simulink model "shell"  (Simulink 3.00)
settings: Solver=ode45  SolverMode=SingleTasking  StartTime=0.0  StopTime=999999  RelTol=1e-3  AbsTol=1e-6
undefined symbols (not defined in the file or in its folder): Manual

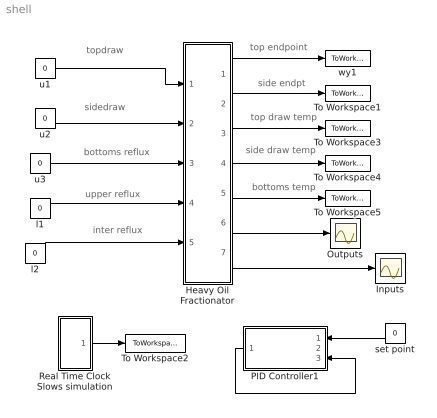
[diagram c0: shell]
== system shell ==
  note: topdraw
  note: sidedraw
  note: bottoms reflux
  note: upper reflux
  note: inter reflux
  note: top endpoint
  note: side endpt
  note: top draw temp
  note: side draw temp
  note: bottoms temp
  Heavy Oil Fractionator : Subsystem  mask{e5=0.0, e4=0.0, e3=0.0, e2=0.0, e1=0.0}
      mask prompts: e5 "Error in Upp Ref Duty Tfns"; e4 "Error in Int Ref Duty Tfns"; e3 "Error in Bott duty tfns"; e2 "Err in Side draw tfns"; e1 "Error in top draw tfs"
      mask init:
      | e1=0;e2=0;e3=0;e4=0;e5=0;
  Inputs : Scope
  Outputs : Scope
  PID Controller1 : Subsystem  Orientation=left  mask(Real PID Controller){am_flag=Manual, co=0, Ts=1, Kc=0, taui=999999, taud=0, co_max=.5, co_min=-.5, al=0}
      mask prompts: am_flag "Auto/Manual Switch"; co "Manual Controller Output"; Ts "Sample Time,Ts"; Kc "Kc: Proportional Gain: Negative for DIRECT Action"; taui "taui: Integral time"; taud "Derivative Time, taud"; co_max "Upper limit for controller output"; co_min "Lower limit for controller output"; al "Noise filter tim const, al"
      mask help: Programmed by Babu Joseph, Washington Universtiy in St. Louis, 1998
  Real Time Clock Slows simulation : Subsystem  mask(Sample time){Ts=1}
      mask prompts: Ts "Sample time"
      mask help: This block is used to set the sample time.
  To Workspace1 : ToWorkspace  VariableName=y2  SampleTime=1  SaveFormat=Matrix
  To Workspace2 : ToWorkspace  VariableName=t  SampleTime=1  SaveFormat=Matrix
  To Workspace3 : ToWorkspace  VariableName=y3  SampleTime=1  SaveFormat=Matrix
  To Workspace4 : ToWorkspace  VariableName=y5  SampleTime=1  SaveFormat=Matrix
  To Workspace5 : ToWorkspace  VariableName=y7  SampleTime=1  SaveFormat=Matrix
  l1 : Constant  Value=0
  l2 : Constant  Value=0
  set point : Constant  Orientation=left  Value=0
  u1 : Constant  Value=0
  u2 : Constant  Value=0
  u3 : Constant  Value=0
  wy1 : ToWorkspace  VariableName=y1  SampleTime=1  SaveFormat=Matrix
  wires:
  u3/1 -> Heavy Oil Fractionator/3(u3)
  l2/1 -> Heavy Oil Fractionator/5(l2)
  l1/1 -> Heavy Oil Fractionator/4(l1)
  Heavy Oil Fractionator/6(outputs) -> Outputs/1
  Heavy Oil Fractionator/7(inputs) -> Inputs/1
  Heavy Oil Fractionator/2(y2) -> To Workspace1/1
  Heavy Oil Fractionator/3(y3) -> To Workspace3/1
  Heavy Oil Fractionator/4(y5) -> To Workspace4/1
  Heavy Oil Fractionator/5(y7) -> To Workspace5/1
  Real Time Clock Slows simulation/1("Clock ") -> To Workspace2/1
  u2/1 -> Heavy Oil Fractionator/2(u2)
  Heavy Oil Fractionator/1(y1) -> wy1/1
  u1/1 -> Heavy Oil Fractionator/1(u1)
  set point/1 -> PID Controller1/1(setpt)
  PID Controller1/1(output) -> PID Controller1/3(out_fdbk)
  ? -> PID Controller1/2(meas)

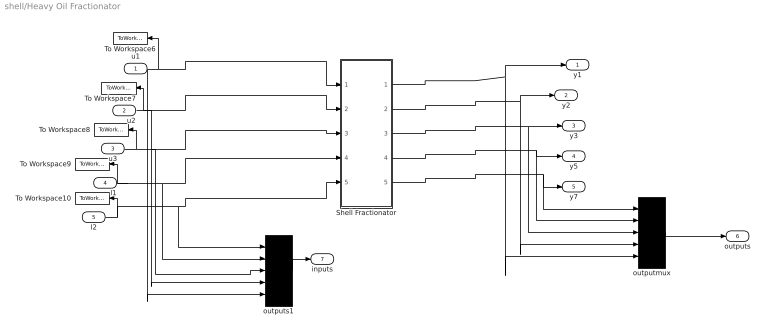
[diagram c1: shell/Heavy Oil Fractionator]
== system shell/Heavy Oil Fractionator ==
  u1 : Inport  Port=1  PortWidth=-1  SampleTime=-1  DataType=auto
  u2 : Inport  Port=2  PortWidth=-1  SampleTime=-1  DataType=auto
  u3 : Inport  Port=3  PortWidth=-1  SampleTime=-1  DataType=auto
  l1 : Inport  Port=4  PortWidth=-1  SampleTime=-1  DataType=auto
  l2 : Inport  Port=5  PortWidth=-1  SampleTime=-1  DataType=auto
  Shell Fractionator : Subsystem
  To Workspace10 : ToWorkspace  VariableName=l2  SampleTime=1  SaveFormat=Matrix
  To Workspace6 : ToWorkspace  VariableName=u1  SampleTime=1  SaveFormat=Matrix
  To Workspace7 : ToWorkspace  VariableName=u2  SampleTime=1  SaveFormat=Matrix
  To Workspace8 : ToWorkspace  VariableName=u3  SampleTime=1  SaveFormat=Matrix
  To Workspace9 : ToWorkspace  VariableName=l1  SampleTime=1  SaveFormat=Matrix
  outputmux : Mux  Inputs=5
  outputs1 : Mux  Inputs=5
  y1 : Outport  Port=1  InitialOutput=0
  y2 : Outport  Port=2  InitialOutput=0
  y3 : Outport  Port=3  InitialOutput=0
  y5 : Outport  Port=4  InitialOutput=0
  y7 : Outport  Port=5  InitialOutput=0
  outputs : Outport  Port=6  InitialOutput=0
  inputs : Outport  Port=7  InitialOutput=0
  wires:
  l2/1 -> To Workspace10/1, outputs1/1, Shell Fractionator/5(l2)
  l1/1 -> To Workspace9/1, outputs1/2, Shell Fractionator/4(l1)
  u3/1 -> To Workspace8/1, outputs1/3, Shell Fractionator/3(u3)
  u2/1 -> To Workspace7/1, outputs1/4, Shell Fractionator/2(u2)
  outputmux/1 -> outputs/1
  outputs1/1 -> inputs/1
  u1/1 -> To Workspace6/1, Shell Fractionator/1(u1), outputs1/5
  Shell Fractionator/1(y1) -> y1/1, outputmux/5
  Shell Fractionator/2(y2) -> y2/1, outputmux/4
  Shell Fractionator/3(y3) -> y3/1, outputmux/3
  Shell Fractionator/4(y5) -> y5/1, outputmux/2
  Shell Fractionator/5(y7) -> y7/1, outputmux/1

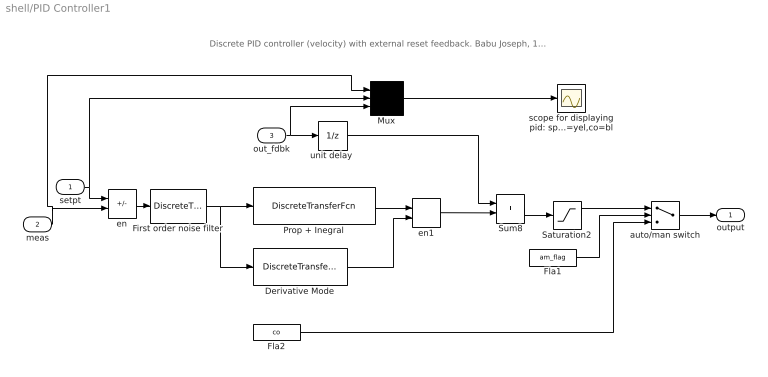
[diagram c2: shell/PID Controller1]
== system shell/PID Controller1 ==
  note: Discrete PID controller (velocity) with external reset feedback. Babu Joseph, 1998
  setpt : Inport  Port=1  PortWidth=-1  SampleTime=-1  DataType=auto
  meas : Inport  Port=2  PortWidth=-1  SampleTime=-1  DataType=auto
  out_fdbk : Inport  Port=3  PortWidth=-1  SampleTime=-1  DataType=auto
  Derivative Mode : DiscreteTransferFcn  Numerator=Kc*taud*[1 -2 1]  Denominator=[ 1 0 0]  SampleTime=Ts
  First order noise filter : DiscreteTransferFcn  Numerator="[Ts   0]"  Denominator="[(al+Ts)  -al]"  SampleTime=Ts
  Fla1 : Constant  Value=am_flag
  Fla2 : Constant  Value=co
  Mux : Mux  Inputs=3
  Prop + Inegral : DiscreteTransferFcn  Numerator="Kc*[ (1+Ts/taui)  -1 ]"  Denominator="[ 1  0 ]"  SampleTime=Ts
  Saturation2 : Saturate  UpperLimit=co_max  LowerLimit=co_min
  Sum8 : Sum  Inputs=++  SaturateOnIntegerOverflow=on
  auto/man switch : Switch  Threshold=1.5
  en : Sum  Inputs=+-  SaturateOnIntegerOverflow=on
  en1 : Sum  Inputs=++  SaturateOnIntegerOverflow=on
  scope for displaying pid: sp=red,mv=yel,co=bl : Scope
  "unit delay " : UnitDelay  X0=co  SampleTime=Ts
  output : Outport  Port=1  InitialOutput=0
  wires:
  meas/1 -> Mux/1, en/2
  Sum8/1 -> Saturation2/1
  Saturation2/1 -> auto/man switch/1
  Fla1/1 -> auto/man switch/2
  Derivative Mode/1 -> en1/2
  en1/1 -> Sum8/2
  setpt/1 -> en/1, Mux/2
  en/1 -> First order noise filter/1
  Fla2/1 -> auto/man switch/3
  auto/man switch/1 -> output/1
  Mux/1 -> scope for displaying pid: sp=red,mv=yel,co=bl/1
  out_fdbk/1 -> Mux/3, "unit delay "/1
  "unit delay "/1 -> Sum8/1
  First order noise filter/1 -> Derivative Mode/1, Prop + Inegral/1
  Prop + Inegral/1 -> en1/1

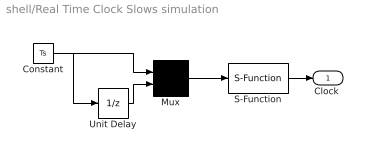
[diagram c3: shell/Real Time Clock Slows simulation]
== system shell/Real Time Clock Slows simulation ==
  Constant : Constant  Value=Ts
  Mux : Mux  Inputs=2
  S-Function : S-Function  FunctionName=wait3  PortCounts=[]  SFunctionModules=''
  Unit Delay : UnitDelay  X0=0  SampleTime=Ts
  "Clock " : Outport  Port=1  InitialOutput=0
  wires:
  S-Function/1 -> "Clock "/1
  Mux/1 -> S-Function/1
  Unit Delay/1 -> Mux/2
  Constant/1 -> Mux/1, Unit Delay/1

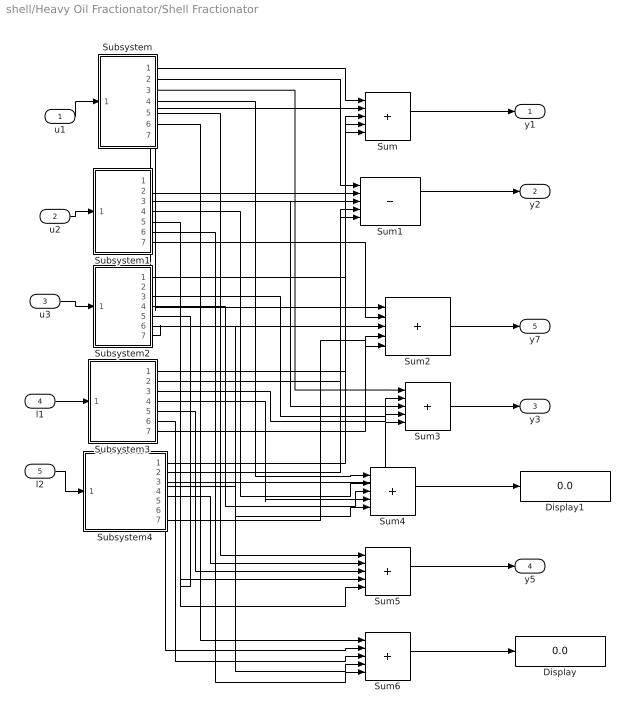
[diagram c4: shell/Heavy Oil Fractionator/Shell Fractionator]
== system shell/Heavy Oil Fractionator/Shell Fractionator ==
  u1 : Inport  Port=1  PortWidth=-1  SampleTime=-1  DataType=auto
  u2 : Inport  Port=2  PortWidth=-1  SampleTime=-1  DataType=auto
  u3 : Inport  Port=3  PortWidth=-1  SampleTime=-1  DataType=auto
  l1 : Inport  Port=4  PortWidth=-1  SampleTime=-1  DataType=auto
  l2 : Inport  Port=5  PortWidth=-1  SampleTime=-1  DataType=auto
  Display : Display
  Display1 : Display
  Subsystem : Subsystem
  Subsystem1 : Subsystem
  Subsystem2 : Subsystem
  Subsystem3 : Subsystem
  Subsystem4 : Subsystem
  Sum{,1..6} (7 alike) : Sum  Inputs=+++++  SaturateOnIntegerOverflow=on
  y1 : Outport  Port=1  InitialOutput=0
  y2 : Outport  Port=2  InitialOutput=0
  y3 : Outport  Port=3  InitialOutput=0
  y5 : Outport  Port=4  InitialOutput=0
  y7 : Outport  Port=5  InitialOutput=0
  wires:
  l2/1 -> Subsystem4/1(In1)
  l1/1 -> Subsystem3/1(In1)
  Sum2/1 -> y7/1
  u3/1 -> Subsystem2/1(In1)
  u2/1 -> Subsystem1/1(In1)
  u1/1 -> Subsystem/1(In1)
  Sum/1 -> y1/1
  Subsystem4/2(Out2) -> Sum1/5
  Subsystem4/1(Out1) -> Sum/5
  Subsystem3/7(Out7) -> Sum2/4
  Subsystem3/2(Out2) -> Sum1/4
  Subsystem3/1(Out1) -> Sum/4
  Subsystem2/2(Out2) -> Sum1/3
  Subsystem2/1(Out1) -> Sum/3
  Subsystem2/7(Out7) -> Sum2/3
  Subsystem1/2(Out2) -> Sum1/2
  Subsystem1/1(Out1) -> Sum/2
  Subsystem/7(Out7) -> Sum2/1
  Subsystem/2(Out2) -> Sum1/1
  Subsystem/1(Out1) -> Sum/1
  Sum1/1 -> y2/1
  Subsystem1/7(Out7) -> Sum2/2
  Sum3/1 -> y3/1
  Sum4/1 -> Display1/1
  Sum5/1 -> y5/1
  Sum6/1 -> Display/1
  Subsystem/3(Out3) -> Sum3/1
  Subsystem1/3(Out3) -> Sum3/2
  Subsystem2/3(Out3) -> Sum3/3
  Subsystem3/3(Out3) -> Sum3/4
  Subsystem4/3(Out3) -> Sum3/5
  Subsystem4/7(Out7) -> Sum2/5
  Subsystem/4(Out4) -> Sum4/1
  Subsystem1/4(Out4) -> Sum4/2
  Subsystem2/4(Out4) -> Sum4/3
  Subsystem3/4(Out4) -> Sum4/4
  Subsystem4/4(Out4) -> Sum4/5
  Subsystem/5("Out5 ") -> Sum5/1
  Subsystem4/5(Out5) -> Sum5/2
  Subsystem3/5(Out5) -> Sum5/3
  Subsystem2/5(Out5) -> Sum5/4
  Subsystem1/5(Out5) -> Sum5/5
  Subsystem/6("Out6 ") -> Sum6/1
  Subsystem4/6(Out6) -> Sum6/2
  Subsystem3/6(Out6) -> Sum6/3
  Subsystem2/6(Out6) -> Sum6/4
  Subsystem1/6(Out6) -> Sum6/5

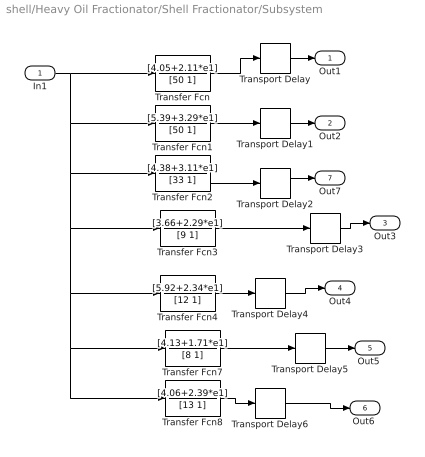
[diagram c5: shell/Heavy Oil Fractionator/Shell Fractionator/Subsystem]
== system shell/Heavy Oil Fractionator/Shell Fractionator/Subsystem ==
  In1 : Inport  Port=1  PortWidth=-1  SampleTime=-1  DataType=auto
  Transfer Fcn : TransferFcn  Numerator=[4.05+2.11*e1]  Denominator=[50 1]
  Transfer Fcn1 : TransferFcn  Numerator=[5.39+3.29*e1]  Denominator=[50 1]
  Transfer Fcn2 : TransferFcn  Numerator=[4.38+3.11*e1]  Denominator=[33 1]
  Transfer Fcn3 : TransferFcn  Numerator=[3.66+2.29*e1]  Denominator=[9 1]
  Transfer Fcn4 : TransferFcn  Numerator=[5.92+2.34*e1]  Denominator=[12 1]
  Transfer Fcn7 : TransferFcn  Numerator=[4.13+1.71*e1]  Denominator=[8 1]
  Transfer Fcn8 : TransferFcn  Numerator=[4.06+2.39*e1]  Denominator=[13 1]
  Transport Delay : TransportDelay  DelayTime=27  InitialInput=0  BufferSize=1024
  Transport Delay1 : TransportDelay  DelayTime=18  InitialInput=0  BufferSize=1024
  Transport Delay2 : TransportDelay  DelayTime=20  InitialInput=0  BufferSize=1024
  Transport Delay3 : TransportDelay  DelayTime=2  InitialInput=0  BufferSize=1024
  Transport Delay4 : TransportDelay  DelayTime=11  InitialInput=0  BufferSize=1024
  Transport Delay5 : TransportDelay  DelayTime=5  InitialInput=0  BufferSize=1024
  Transport Delay6 : TransportDelay  DelayTime=8  InitialInput=0  BufferSize=1024
  Out1 : Outport  Port=1  InitialOutput=0
  Out2 : Outport  Port=2  InitialOutput=0
  Out3 : Outport  Port=3  InitialOutput=0
  Out4 : Outport  Port=4  InitialOutput=0
  "Out5 " : Outport  Port=5  InitialOutput=0
  "Out6 " : Outport  Port=6  InitialOutput=0
  Out7 : Outport  Port=7  InitialOutput=0
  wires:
  Transport Delay2/1 -> Out7/1
  Transport Delay1/1 -> Out2/1
  Transfer Fcn2/1 -> Transport Delay2/1
  Transfer Fcn1/1 -> Transport Delay1/1
  In1/1 -> Transfer Fcn1/1, Transfer Fcn2/1, Transfer Fcn3/1, Transfer Fcn4/1, Transfer Fcn7/1, Transfer Fcn8/1, Transfer Fcn/1
  Transfer Fcn3/1 -> Transport Delay3/1
  Transfer Fcn4/1 -> Transport Delay4/1
  Transfer Fcn7/1 -> Transport Delay5/1
  Transport Delay4/1 -> Out4/1
  Transport Delay5/1 -> "Out5 "/1
  Transfer Fcn8/1 -> Transport Delay6/1
  Transport Delay6/1 -> "Out6 "/1
  Transport Delay3/1 -> Out3/1
  Transport Delay/1 -> Out1/1
  Transfer Fcn/1 -> Transport Delay/1

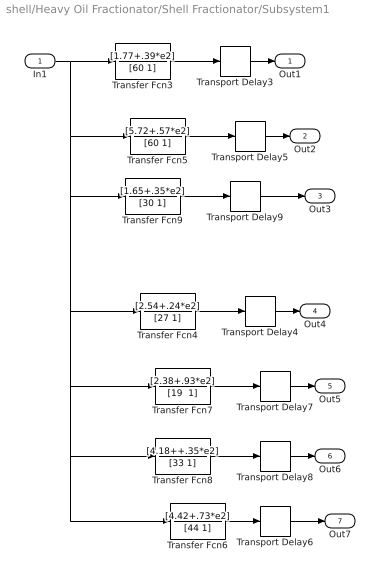
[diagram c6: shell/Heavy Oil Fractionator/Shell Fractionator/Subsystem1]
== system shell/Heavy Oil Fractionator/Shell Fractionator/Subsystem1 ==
  In1 : Inport  Port=1  PortWidth=-1  SampleTime=-1  DataType=auto
  Transfer Fcn3 : TransferFcn  Numerator=[1.77+.39*e2]  Denominator=[60 1]
  Transfer Fcn4 : TransferFcn  Numerator=[2.54+.24*e2]  Denominator=[27 1]
  Transfer Fcn5 : TransferFcn  Numerator=[5.72+.57*e2]  Denominator=[60 1]
  Transfer Fcn6 : TransferFcn  Numerator=[4.42+.73*e2]  Denominator=[44 1]
  Transfer Fcn7 : TransferFcn  Numerator=[2.38+.93*e2]  Denominator="[19  1]"
  Transfer Fcn8 : TransferFcn  Numerator=[4.18++.35*e2]  Denominator=[33 1]
  Transfer Fcn9 : TransferFcn  Numerator=[1.65+.35*e2]  Denominator=[30 1]
  Transport Delay3 : TransportDelay  DelayTime=28  InitialInput=0  BufferSize=1024
  Transport Delay4 : TransportDelay  DelayTime=12  InitialInput=0  BufferSize=1024
  Transport Delay5 : TransportDelay  DelayTime=14  InitialInput=0  BufferSize=1024
  Transport Delay6 : TransportDelay  DelayTime=22  InitialInput=0  BufferSize=1024
  Transport Delay7 : TransportDelay  DelayTime=7  InitialInput=0  BufferSize=1024
  Transport Delay8 : TransportDelay  DelayTime=4  InitialInput=0  BufferSize=1024
  Transport Delay9 : TransportDelay  DelayTime=20  InitialInput=0  BufferSize=1024
  Out1 : Outport  Port=1  InitialOutput=0
  Out2 : Outport  Port=2  InitialOutput=0
  Out3 : Outport  Port=3  InitialOutput=0
  Out4 : Outport  Port=4  InitialOutput=0
  Out5 : Outport  Port=5  InitialOutput=0
  Out6 : Outport  Port=6  InitialOutput=0
  Out7 : Outport  Port=7  InitialOutput=0
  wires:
  Transport Delay5/1 -> Out2/1
  Transport Delay3/1 -> Out1/1
  In1/1 -> Transfer Fcn5/1, Transfer Fcn6/1, Transfer Fcn4/1, Transfer Fcn7/1, Transfer Fcn8/1, Transfer Fcn9/1, Transfer Fcn3/1
  Transfer Fcn5/1 -> Transport Delay5/1
  Transfer Fcn3/1 -> Transport Delay3/1
  Transport Delay8/1 -> Out6/1
  Transport Delay7/1 -> Out5/1
  Transport Delay4/1 -> Out4/1
  Transfer Fcn8/1 -> Transport Delay8/1
  Transfer Fcn7/1 -> Transport Delay7/1
  Transfer Fcn4/1 -> Transport Delay4/1
  Transport Delay9/1 -> Out3/1
  Transfer Fcn9/1 -> Transport Delay9/1
  Transport Delay6/1 -> Out7/1
  Transfer Fcn6/1 -> Transport Delay6/1

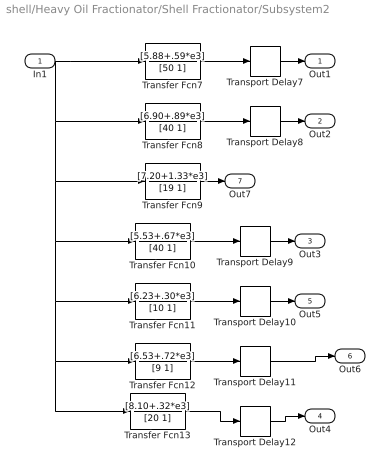
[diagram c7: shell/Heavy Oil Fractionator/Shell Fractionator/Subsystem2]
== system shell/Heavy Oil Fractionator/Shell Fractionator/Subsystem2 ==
  In1 : Inport  Port=1  PortWidth=-1  SampleTime=-1  DataType=auto
  Transfer Fcn10 : TransferFcn  Numerator=[5.53+.67*e3]  Denominator=[40 1]
  Transfer Fcn11 : TransferFcn  Numerator=[6.23+.30*e3]  Denominator=[10 1]
  Transfer Fcn12 : TransferFcn  Numerator=[6.53+.72*e3]  Denominator=[9 1]
  Transfer Fcn13 : TransferFcn  Numerator=[8.10+.32*e3]  Denominator=[20 1]
  Transfer Fcn7 : TransferFcn  Numerator=[5.88+.59*e3]  Denominator=[50 1]
  Transfer Fcn8 : TransferFcn  Numerator=[6.90+.89*e3]  Denominator=[40 1]
  Transfer Fcn9 : TransferFcn  Numerator=[7.20+1.33*e3]  Denominator=[19 1]
  Transport Delay10 : TransportDelay  DelayTime=2  InitialInput=0  BufferSize=1024
  Transport Delay11 : TransportDelay  DelayTime=1  InitialInput=0  BufferSize=1024
  Transport Delay12 : TransportDelay  DelayTime=2  InitialInput=0  BufferSize=1024
  Transport Delay7 : TransportDelay  DelayTime=27  InitialInput=0  BufferSize=1024
  Transport Delay8 : TransportDelay  DelayTime=15  InitialInput=0  BufferSize=1024
  Transport Delay9 : TransportDelay  DelayTime=2  InitialInput=0  BufferSize=1024
  Out1 : Outport  Port=1  InitialOutput=0
  Out2 : Outport  Port=2  InitialOutput=0
  Out3 : Outport  Port=3  InitialOutput=0
  Out4 : Outport  Port=4  InitialOutput=0
  Out5 : Outport  Port=5  InitialOutput=0
  Out6 : Outport  Port=6  InitialOutput=0
  Out7 : Outport  Port=7  InitialOutput=0
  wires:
  Transfer Fcn9/1 -> Out7/1
  Transport Delay8/1 -> Out2/1
  Transport Delay7/1 -> Out1/1
  Transfer Fcn8/1 -> Transport Delay8/1
  In1/1 -> Transfer Fcn8/1, Transfer Fcn9/1, Transfer Fcn10/1, Transfer Fcn11/1, Transfer Fcn12/1, Transfer Fcn13/1, Transfer Fcn7/1
  Transfer Fcn7/1 -> Transport Delay7/1
  Transport Delay10/1 -> Out5/1
  Transport Delay9/1 -> Out3/1
  Transfer Fcn11/1 -> Transport Delay10/1
  Transfer Fcn10/1 -> Transport Delay9/1
  Transport Delay11/1 -> Out6/1
  Transfer Fcn12/1 -> Transport Delay11/1
  Transport Delay12/1 -> Out4/1
  Transfer Fcn13/1 -> Transport Delay12/1

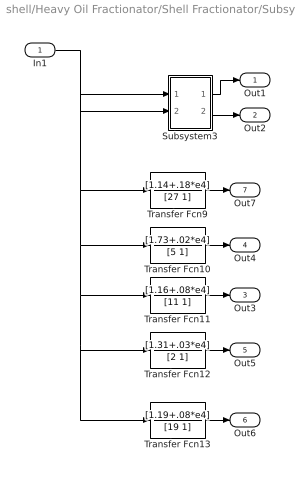
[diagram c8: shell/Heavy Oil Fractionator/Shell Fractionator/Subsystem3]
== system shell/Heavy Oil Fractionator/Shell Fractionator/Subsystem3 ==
  In1 : Inport  Port=1  PortWidth=-1  SampleTime=-1  DataType=auto
  Subsystem3 : Subsystem
  Transfer Fcn10 : TransferFcn  Numerator=[1.73+.02*e4]  Denominator=[5 1]
  Transfer Fcn11 : TransferFcn  Numerator=[1.16+.08*e4]  Denominator=[11 1]
  Transfer Fcn12 : TransferFcn  Numerator=[1.31+.03*e4]  Denominator=[2 1]
  Transfer Fcn13 : TransferFcn  Numerator=[1.19+.08*e4]  Denominator=[19 1]
  Transfer Fcn9 : TransferFcn  Numerator=[1.14+.18*e4]  Denominator=[27 1]
  Out1 : Outport  Port=1  InitialOutput=0
  Out2 : Outport  Port=2  InitialOutput=0
  Out3 : Outport  Port=3  InitialOutput=0
  Out4 : Outport  Port=4  InitialOutput=0
  Out5 : Outport  Port=5  InitialOutput=0
  Out6 : Outport  Port=6  InitialOutput=0
  Out7 : Outport  Port=7  InitialOutput=0
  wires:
  Subsystem3/1(Out1) -> Out1/1
  In1/1 -> Subsystem3/1(In1), Subsystem3/2(In2), Transfer Fcn9/1, Transfer Fcn10/1, Transfer Fcn11/1, Transfer Fcn12/1, Transfer Fcn13/1
  Transfer Fcn9/1 -> Out7/1
  Transfer Fcn10/1 -> Out4/1
  Transfer Fcn11/1 -> Out3/1
  Transfer Fcn12/1 -> Out5/1
  Transfer Fcn13/1 -> Out6/1
  Subsystem3/2(Out2) -> Out2/1

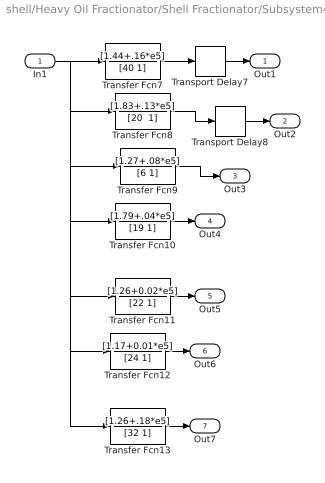
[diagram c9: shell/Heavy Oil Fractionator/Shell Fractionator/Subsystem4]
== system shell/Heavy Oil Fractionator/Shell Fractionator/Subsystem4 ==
  In1 : Inport  Port=1  PortWidth=-1  SampleTime=-1  DataType=auto
  Transfer Fcn10 : TransferFcn  Numerator=[1.79+.04*e5]  Denominator=[19 1]
  Transfer Fcn11 : TransferFcn  Numerator=[1.26+0.02*e5]  Denominator=[22 1]
  Transfer Fcn12 : TransferFcn  Numerator=[1.17+0.01*e5]  Denominator=[24 1]
  Transfer Fcn13 : TransferFcn  Numerator=[1.26+.18*e5]  Denominator=[32 1]
  Transfer Fcn7 : TransferFcn  Numerator=[1.44+.16*e5]  Denominator=[40 1]
  Transfer Fcn8 : TransferFcn  Numerator=[1.83+.13*e5]  Denominator="[20  1]"
  Transfer Fcn9 : TransferFcn  Numerator=[1.27+.08*e5]  Denominator=[6 1]
  Transport Delay7 : TransportDelay  DelayTime=27  InitialInput=0  BufferSize=1024
  Transport Delay8 : TransportDelay  DelayTime=15  InitialInput=0  BufferSize=1024
  Out1 : Outport  Port=1  InitialOutput=0
  Out2 : Outport  Port=2  InitialOutput=0
  Out3 : Outport  Port=3  InitialOutput=0
  Out4 : Outport  Port=4  InitialOutput=0
  Out5 : Outport  Port=5  InitialOutput=0
  Out6 : Outport  Port=6  InitialOutput=0
  Out7 : Outport  Port=7  InitialOutput=0
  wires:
  Transfer Fcn9/1 -> Out3/1
  Transport Delay8/1 -> Out2/1
  Transport Delay7/1 -> Out1/1
  In1/1 -> Transfer Fcn8/1, Transfer Fcn9/1, Transfer Fcn10/1, Transfer Fcn11/1, Transfer Fcn13/1, Transfer Fcn12/1, Transfer Fcn7/1
  Transfer Fcn8/1 -> Transport Delay8/1
  Transfer Fcn7/1 -> Transport Delay7/1
  Transfer Fcn10/1 -> Out4/1
  Transfer Fcn11/1 -> Out5/1
  Transfer Fcn12/1 -> Out6/1
  Transfer Fcn13/1 -> Out7/1

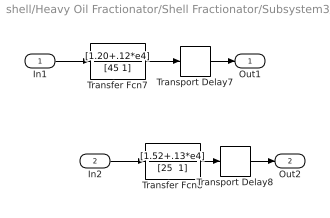
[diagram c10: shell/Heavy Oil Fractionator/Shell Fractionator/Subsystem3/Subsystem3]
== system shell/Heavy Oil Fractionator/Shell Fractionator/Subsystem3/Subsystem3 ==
  In1 : Inport  Port=1  PortWidth=-1  SampleTime=-1  DataType=auto
  In2 : Inport  Port=2  PortWidth=-1  SampleTime=-1  DataType=auto
  Transfer Fcn7 : TransferFcn  Numerator=[1.20+.12*e4]  Denominator=[45 1]
  Transfer Fcn8 : TransferFcn  Numerator=[1.52+.13*e4]  Denominator="[25  1]"
  Transport Delay7 : TransportDelay  DelayTime=27  InitialInput=0  BufferSize=1024
  Transport Delay8 : TransportDelay  DelayTime=15  InitialInput=0  BufferSize=1024
  Out1 : Outport  Port=1  InitialOutput=0
  Out2 : Outport  Port=2  InitialOutput=0
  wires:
  Transport Delay8/1 -> Out2/1
  Transport Delay7/1 -> Out1/1
  In2/1 -> Transfer Fcn8/1
  In1/1 -> Transfer Fcn7/1
  Transfer Fcn8/1 -> Transport Delay8/1
  Transfer Fcn7/1 -> Transport Delay7/1
